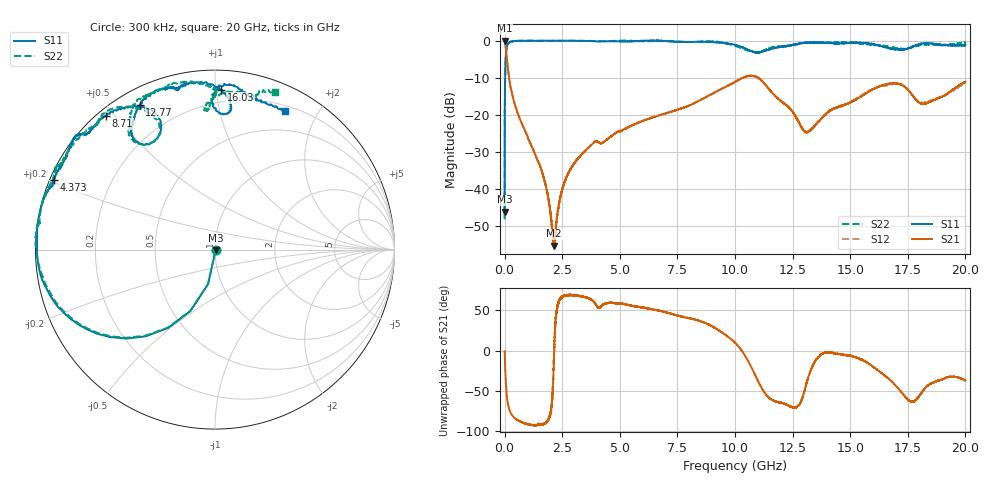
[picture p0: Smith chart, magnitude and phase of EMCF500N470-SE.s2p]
!EMCF500N470
!Johanson Technology Inc.
!www.johansontechnology.com
!Test Board Conditions:
!Substrate Type  RO4350B
!Substrate Thickness  6.6 mil
!Substrate Dk  3.66
!TL Type: GCPW
!TL Trace Width  13 mil
!TL Gap  7.5 mil
!PART MODE SINGLE ENDED (AKA BYPASS)
!DUT TOPOLOGY	SERIES-SHUNT
# MHz S  dB  R 50
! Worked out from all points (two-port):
!   20001 points, 300 kHz to 20 GHz, reference 50 ohm
!   highest |S21| = 0.02 dB at 300 kHz (marker M1); lowest = -55.3 dB at 2.148 GHz (marker M2)
!   |S21| within 3 dB of the highest: start of sweep to 65.4 MHz
!   lowest |S11| = -46.1 dB at 300 kHz (marker M3), VSWR 1.01, Z = 50.3 - j0.356 ohm
!   |S11| at or under -10 dB: start of sweep to 22.15 MHz
!   |S22| runs from -48.1 to 0.0 dB; largest |S21 - S12| = 0.015
!   S11 on the Smith chart (normalised r, x): 300 kHz: 1.01, -0.01; 4.373 GHz: 0.01, +0.21; 8.71 GHz: 0.02, +0.47; 12.77 GHz: 0.06, +0.61; 16.03 GHz: 0.12, +1.03; 20 GHz: 0.25, +1.59
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0.3  -46.08 -45.4  0.02 -0.5  0.03 -0.5  -48.11 -41.9
102.298  -1.54 -147.8  -5.35 -57.6  -5.32 -57.6  -1.59 -147.9
170.297  -0.63 -160.0  -8.91 -69.5  -8.87 -69.5  -0.69 -160.0
519.292  -0.10 -175.7  -18.67 -85.2  -18.67 -85.5  -0.08 -177.2
1696.275  -0.03 173.5  -36.89 -90.7  -36.82 -90.5  -0.07 171.9
2148.268  -0.02 169.0  -55.26 -5.9  -54.90 -1.4  -0.09 171.3
2578.261  -0.03 165.6  -38.53 68.1  -38.47 67.7  -0.05 169.3
3334.25  -0.06 161.9  -30.73 67.5  -30.74 67.4  -0.03 162.8
4373.234  -0.19 156.7  -26.97 58.4  -26.92 58.5  -0.12 155.6
6667.2  -0.01 140.5  -20.23 50.0  -20.20 49.8  -0.12 145.7
8710.169  -0.34 129.2  -15.31 34.4  -15.37 34.2  -0.17 130.9
10000.15  -1.17 115.8  -11.15 10.1  -10.96 10.1  -1.42 116.1
11003.14  -3.19 120.5  -9.98 -37.7  -10.11 -38.0  -3.18 121.9
11719.12  -2.01 125.7  -14.73 -62.3  -14.72 -61.4  -1.78 126.0
12769.11  -0.82 117.4  -21.97 -67.5  -21.86 -67.5  -0.85 121.0
13334.1  -0.53 109.3  -23.75 -21.4  -23.69 -21.5  -0.54 115.4
14166.09  -0.67 103.8  -18.69 -2.1  -18.78 -2.4  -0.53 110.2
16032.06  -1.01 87.8  -12.97 -20.8  -12.92 -22.1  -1.15 89.7
16667.05  -2.04 83.6  -11.64 -34.4  -11.96 -34.7  -1.61 91.0
17618.04  -1.87 90.7  -14.04 -62.7  -14.00 -61.7  -1.98 93.4
18177.03  -0.75 86.9  -17.02 -48.9  -16.75 -48.9  -1.10 84.4
20000  -1.23 63.4  -11.08 -36.8  -11.32 -34.8  -0.53 69.0
